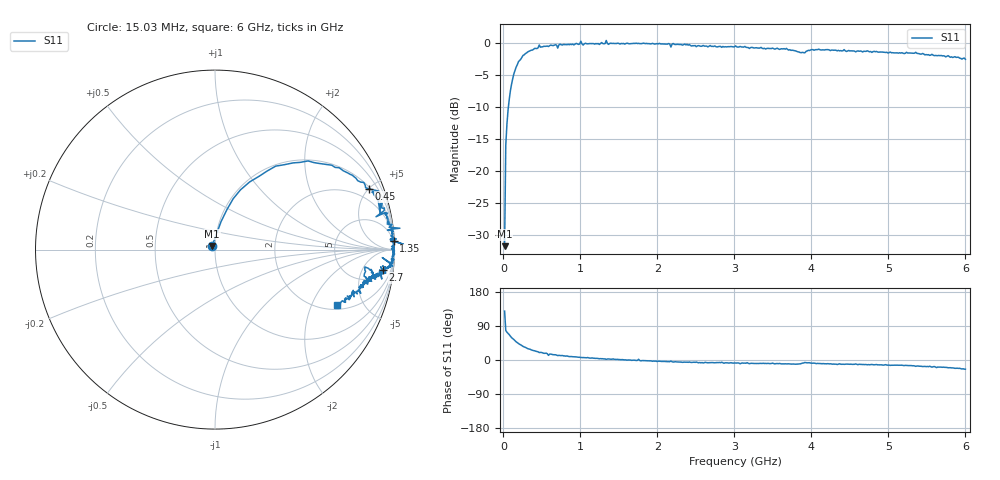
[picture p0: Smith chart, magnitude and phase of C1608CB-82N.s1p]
!	Network	Analyzer	HP8753E.07.74:	Oct	30	2002	Serial	No.	JP38451487
!	Hewlett-Packard
!	7	Sep	2009	9:51:43
!	Frequency	S11
#	HZ	S	RI	R	50
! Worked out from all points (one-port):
!   400 points, 15.03 MHz to 6 GHz, reference 50 ohm
!   lowest |S11| = -31.8 dB at 15.03 MHz (marker M1), VSWR 1.05, Z = 48.4 + j1.94 ohm
!   |S11| at or under -10 dB: start of sweep to 64.14 MHz
!   S11 on the Smith chart (normalised r, x): 15.03 MHz: 0.97, +0.04; 450 MHz: 1.12, +5.00; 1.35 GHz: 4, +43; 2.7 GHz: 7, -14; 6 GHz: 2.26, -3.14
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1.502992e7  -0.0162 0.02
3.002985e7  0.0334 0.155
6.00297e7  0.101 0.283
9.002955e7  0.193 0.377
1.650292e8  0.435 0.483
2.550287e8  0.651 0.47
4.500278e8  0.856 0.339
4.650277e8  0.912 0.326
5.550272e8  0.899 0.294
5.850271e8  0.92 0.2
6.150269e8  0.931 0.259
7.650262e8  0.947 0.2
9.750251e8  0.97 0.124
1.005025e9  1.03 0.119
1.035025e9  0.961 0.108
1.320023e9  0.992 0.0509
1.335023e9  1.05 0.0298
1.350023e9  0.995 0.0458
1.515022e9  0.984 0.0172
1.755021e9  0.996 0.0328
2.265019e9  0.976 -0.0879
2.700016e9  0.937 -0.113
3.015015e9  0.944 -0.132
3.765011e9  0.863 -0.161
3.91501e9  0.835 -0.0965
4.515007e9  0.856 -0.166
5.265004e9  0.811 -0.213
6e9  0.682 -0.307
